[IBIS Ver]   3.2
[File Name]   sprm117a.ibs
[File Rev]   0.2
[Date]   April 12, 2004
[Source]   File Originated at Texas Instruments
[Disclaimer]   Please be aware that in the absence of a written agreement
|   Texas Instruments(TI) assumes no liability for:
|   (1) The accuracy of the IBIS models provided to your company
|   (2) The proper functioning of these Models in your design
|   or for any resulting applications;or
|   (3) Infringement of patents,copyrights, or intellectual
|   property rights resulting from your use of these models.
|   TI provides IBIS Models as a service to our customers and
|   therefore reserves the right to limit distribution of the
|   Models.
[Copyright]   Property of Texas Instruments Incorporated.
|   Unauthorized reproduction and/or distribution is strictly
|   prohibited.
|   This product is protected under copyright law and trade
|   secret law as an unpublished work.
|   Created 1999,(C) Copyright 1999-2000,
|   Texas Instruments Incorporated., All Rights Reserved.
|   These commodities are under the U.S.
|   Government distribution license control.As such,they are not
|   to be re-exported without the prior approval of the U.S.
|   Department of Commerce.
[Notes]   Includes package and IO buffer models for 1.1 and 2.0 SI.
|   REVISION HISTORY
|  Update for April 12, 2004
|   The package model and IBIS models included in this file (sprm117a)
|   apply to TMS silicon for both silcon revision 1.1 and silicon
|   revision 2.0.
|   The package model and IBIS models included in sprm117a are unchanged
|   from those models provided in sprm117.
[Component]   c6411_GLZ
[Manufacturer]   Texas Instruments
[Package]
|Variable   Typ   Min   Max
R_pkg		2.212e-01	1.101e-01	3.279e-01
L_pkg		4.011e-09	2.375e-09	5.798e-09
C_pkg		6.351e-13	3.910e-13	9.306e-13
[Pin] signal_name		model_name	R_pin		L_pin		C_pin
| Clock/PLL Configuration Section
   H4   CLKIN   IDH09_PE100   1.801e-01	3.100e-09	6.130e-13
  AE6	CLKOUT4_GP1	  IDH04_UOT335_PE100	2.381e-01	4.630e-09	6.473e-13
  AD6	CLKOUT6_GP2	  IDH04_UOT335_PE100	2.343e-01	3.341e-09	7.539e-13
   G1   RSV   NC   NA   NA   NA
   H2	  CLKMODE0   IDH09_PE100   2.283e-01	3.995e-09	6.603e-13
| JTAG Emulation Section
 AB16   TMS   IDH09_PS100   1.377e-01	2.655e-09	4.925e-13
 AE19   TDO   IDH04_OUK83_PS100	2.511e-01	4.874e-09	6.498e-13
 AF18   TDI   IDH09_PS100   2.614e-01	5.224e-09	6.920e-13
 AF16   TCLK   IDH09_PS100   2.614e-01	5.224e-09	6.920e-13
 AB15   nTRST   IDH09_PE100   2.614e-01	5.224e-09	6.920e-13
 AE18   EMU9	  IDH04_UOT335_PS100	2.477e-01	4.401e-09	6.871e-13
 AC17   EMU8	  IDH04_UOT335_PS100	1.709e-01	3.536e-09	5.334e-13
 AF17   EMU7	  IDH04_UOT335_PS100	2.500e-01	5.062e-09	6.512e-13
 AD17   EMU6	  IDH04_UOT335_PS100	1.890e-01	3.826e-09	4.936e-13
 AE17   EMU5	  IDH04_UOT335_PS100	2.341e-01	4.430e-09	6.507e-13
 AC16   EMU4	  IDH04_UOT335_PS100	1.551e-01	2.968e-09	5.512e-13
 AD16   EMU3	  IDH04_UOT335_PS100	1.987e-01	3.671e-09	6.373e-13
 AE16   EMU2	  IDH04_UOT335_PS100	2.124e-01	3.853e-09	6.090e-13
 AC15   EMU1	  IDH04_UOT335_PS100	1.646e-01	3.085e-09	5.799e-13
 AF15   EMU0	  IDH04_UOT335_PS100	2.591e-01	4.625e-09	6.938e-13
 AC18   EMU11	  IDH04_UOT335_PS100	1.860e-01	3.449e-09	5.618e-13
 AD18   EMU10	  IDH04_UOT335_PS100	2.025e-01	3.878e-09	5.902e-13
| Resets, Interrupts, and General-Purpose IOs
  AC7   nRESET   IDH09	2.025e-01	3.878e-09	5.902e-13
   B4   NMI   IDH09_PE100   2.697e-01	4.485e-09	7.472e-13
  AF4	GP7_EXTINT7   IDH04_OUK83_PS100	2.697e-01	4.485e-09	7.472e-13
  AD5	GP6_EXTINT6   IDH04_OUK83_PS100	2.697e-01	4.485e-09	7.472e-13
  AE5	GP5_EXTINT5   IDH04_OUK83_PS100	2.697e-01	4.485e-09	7.472e-13
  AF5	GP4_EXTINT4   IDH04_OUK83_PS100	2.697e-01	4.485e-09	7.472e-13
   G3	GP15_nPRST   IDI01_OUG8B	2.697e-01	4.485e-09	7.472e-13
   F2	 GP14_PCLK   IDI01_OUG8B	2.546e-01	4.449e-09	7.097e-13
   G4	GP13_nPINTA   IDI01_OUG8B	2.546e-01	4.449e-09	7.097e-13
   J3	GP12_nPGNT   IDI01_OUG8B	2.546e-01	4.449e-09	7.097e-13
   F1	GP11_nPREQ   IDI01_OUG8B	2.546e-01	4.449e-09	7.097e-13
   L2	GP10_nPCBE3   IDI01_OUG8B	2.546e-01	4.449e-09	7.097e-13
   M3	GP9_PIDSEL   IDI01_OUG8B	1.917e-01	3.882e-09	5.354e-13
  AC6   GP3   IDH04_OUK83_PE100	1.851e-01	3.359e-09	6.075e-13
  AF6   GP0   IDH04_OUK83_PE100	2.922e-01	4.494e-09	8.253e-13
  AE4   GP8   IDH04_OUK83_PE100	2.815e-01	4.759e-09	7.525e-13
| Host-Port Interface (HPI) and Peripheral Component Interconnect (PCI)
  AA4   PCIEN   IDH09_PE100   2.922e-01	4.494e-09	8.253e-13
   R4	nHINT_nPFRAME   IDI01_OUG8B	2.922e-01	4.494e-09	8.253e-13
   R1	HCNTL1_nPDEVSEL   IDI01_OUG8B	2.602e-01	4.276e-09	7.238e-13
   T4	HCNTL0_nPSTOP   IDI01_OUG8B	1.544e-01	3.008e-09	5.439e-13
   R3	HHWIL_nPTRDY   IDI01_OUG8B	1.544e-01	3.008e-09	5.439e-13
   P1	HR/nW_nPCBE2   IDI01_OUG8B	1.544e-01	3.008e-09	5.439e-13
   T3	 nHAS_PPAR   IDI01_OUG8B	1.544e-01	3.008e-09	5.439e-13
   R2	nHCS_nPPERR   IDI01_OUG8B	1.544e-01	3.008e-09	5.439e-13
   T1	nHDS1_nPSERR   IDI01_OUG8B	1.544e-01	3.008e-09	5.439e-13
   T2	nHDS2_nPCBE1   IDI01_OUG8B	1.544e-01	3.008e-09	5.439e-13
   P4	nHRDY_nPIRDY   IDI01_OUG8B	1.432e-01	2.812e-09	4.868e-13
   J2	 HD31_AD31   IDI01_OUG8B	2.239e-01	3.881e-09	6.413e-13
   K3	 HD30_AD30   IDI01_OUG8B	2.011e-01	3.696e-09	5.567e-13
   J1	 HD29_AD29   IDI01_OUG8B	2.725e-01	4.920e-09	7.166e-13
   K4	 HD28_AD28   IDI01_OUG8B	1.590e-01	3.038e-09	5.268e-13
   K2	 HD27_AD27   IDI01_OUG8B	2.196e-01	4.083e-09	6.214e-13
   L3	 HD26_AD26   IDI01_OUG8B	1.822e-01	3.378e-09	5.755e-13
   K1	 HD25_AD25   IDI01_OUG8B	2.676e-01	5.238e-09	6.857e-13
   L4	 HD24_AD24   IDI01_OUG8B	1.692e-01	3.003e-09	5.620e-13
   L1	 HD23_AD23   IDI01_OUG8B	2.646e-01	4.791e-09	6.858e-13
   M4	 HD22_AD22   IDI01_OUG8B	1.455e-01	2.797e-09	5.032e-13
   M2	 HD21_AD21   IDI01_OUG8B	2.098e-01	3.830e-09	5.948e-13
   N4	 HD20_AD20   IDI01_OUG8B	1.611e-01	2.974e-09	5.102e-13
   M1	 HD19_AD19   IDI01_OUG8B	2.475e-01	4.493e-09	6.660e-13
   N5	 HD18_AD18   IDI01_OUG8B	1.114e-01	2.452e-09	4.378e-13
   N1	 HD17_AD17   IDI01_OUG8B	2.536e-01	4.462e-09	6.731e-13
   P5	 HD16_AD16   IDI01_OUG8B	1.387e-01	2.604e-09	5.119e-13
   U4	 HD15_AD15   IDI01_OUG8B	1.709e-01	3.367e-09	5.453e-13
   U1	 HD14_AD14   IDI01_OUG8B	2.504e-01	4.977e-09	6.598e-13
   U3	 HD13_AD13   IDI01_OUG8B	1.886e-01	3.777e-09	4.994e-13
   U2	 HD12_AD12   IDI01_OUG8B	2.321e-01	4.441e-09	6.047e-13
   V4	 HD11_AD11   IDI01_OUG8B	1.869e-01	3.381e-09	5.890e-13
   V1	 HD10_AD10   IDI01_OUG8B	2.598e-01	5.197e-09	6.873e-13
   V3	 HD09_AD09   IDI01_OUG8B	2.598e-01	5.197e-09	6.873e-13
   V2	 HD08_AD08   IDI01_OUG8B	2.598e-01	5.197e-09	6.873e-13
   W2	 HD07_AD07   IDI01_OUG8B	2.598e-01	5.197e-09	6.873e-13
   W4	 HD06_AD06   IDI01_OUG8B	2.598e-01	5.197e-09	6.873e-13
   Y1	 HD05_AD05   IDI01_OUG8B	2.598e-01	5.197e-09	6.873e-13
   Y3	 HD04_AD04   IDI01_OUG8B	2.598e-01	5.197e-09	6.873e-13
   Y2	 HD03_AD03   IDI01_OUG8B	2.598e-01	5.197e-09	6.873e-13
   Y4	 HD02_AD02   IDI01_OUG8B	2.598e-01	5.197e-09	6.873e-13
  AA1	 HD01_AD01   IDI01_OUG8B	2.598e-01	5.197e-09	6.873e-13
  AA3	 HD00_AD00   IDI01_OUG8B	2.598e-01	5.197e-09	6.873e-13
   W3   nPCBE0   IDI01_OUG8B	2.598e-01	5.197e-09	6.873e-13
  AD1   XSPCS   IDH04_OUK83_PE100	2.598e-01	5.197e-09	6.873e-13
  AC2   XSPCLK   IDH04_OUK83_PE100	2.690e-01	4.510e-09	7.463e-13
  AB3   XSPDI   IDH04_PS100	2.430e-01	4.177e-09	6.584e-13
  AA2   XSPDO   IDH04_OUK83_PS100	2.703e-01	4.736e-09	7.142e-13
| EMIF Control Signals
  L26   nCE3	  IDH04_UOT335_PS100	2.598e-01	5.197e-09	6.873e-13
  K23   nCE2	  IDH04_UOT335_PS100	2.598e-01	5.197e-09	6.873e-13
  K24   nCE1	  IDH04_UOT335_PS100	2.598e-01	5.197e-09	6.873e-13
  K25   nCE0	  IDH04_UOT335_PS100	2.598e-01	5.197e-09	6.873e-13
  T23   RSV   NC   NA   NA   NA
  T24   RSV   NC   NA   NA   NA
  R25   RSV   NC   NA   NA   NA
  R26   RSV   NC   NA   NA   NA
  M25   nBE03	  IDH04_UOT335_PS100	2.598e-01	5.197e-09	6.873e-13
  M26   nBE02	  IDH04_UOT335_PS100	2.598e-01	5.197e-09	6.873e-13
  L23   nBE01	  IDH04_UOT335_PS100	2.598e-01	5.197e-09	6.873e-13
  L24   nBE00	  IDH04_UOT335_PS100	2.598e-01	5.197e-09	6.873e-13
  M22   nPDT	  IDH04_UOT335_PS100	2.598e-01	5.197e-09	6.873e-13
| EMIF Bus Arbitration
  N22   nHOLDA	  IDH04_UOT335_PS100	2.598e-01	5.197e-09	6.873e-13
  V23   nHOLD   IDH09_PS100   2.598e-01	5.197e-09	6.873e-13
  P22	  BUSREQ0	  IDH04_UOT335_PS100	2.598e-01	5.197e-09	6.873e-13
| EMIF Async/Sync Memory Control
  H25   ECLKIN   IDH09_PE100   2.511e-01	4.592e-09	6.768e-13
  J23	 ECLKOUT2	  IDH04_UOT335_PE100	1.851e-01	3.434e-09	5.608e-13
  J26	 ECLKOUT1	  IDH04_UOT335_PE100	2.599e-01	5.229e-09	6.780e-13
  J25   nSDCAS	  IDH04_UOT335_PS100	2.467e-01	4.341e-09	6.879e-13
  J24   nSDRAS	  IDH04_UOT335_PS100	2.014e-01	3.844e-09	5.854e-13
  K26   nSDWE	  IDH04_UOT335_PS100	2.494e-01	5.112e-09	6.385e-13
  L25   SDCKE	  IDH04_UOT335_PS100	2.118e-01	3.884e-09	5.955e-13
  R22   nSOE3	  IDH04_UOT335_PS100	2.118e-01	3.884e-09	5.955e-13
  L22   ARDY   IDH09_PS100   1.370e-01	2.710e-09	4.841e-13
| EMIF Address
  T22   EA22	  IDH04_UOT335_PE100	1.229e-01	2.684e-09	4.276e-13
  V24   EA21	  IDH04_UOT335_PE100	2.064e-01	3.768e-09	6.312e-13
  V25   EA20	  IDH04_UOT335_PE100	2.195e-01	4.186e-09	6.132e-13
  V26   EA19	  IDH04_UOT335_PE100	2.732e-01	4.782e-09	7.055e-13
  U23   EA18	  IDH04_UOT335_PE100	1.584e-01	2.852e-09	5.393e-13
  U24   EA17	  IDH04_UOT335_PE100	2.008e-01	3.829e-09	5.212e-13
  U25   EA16	  IDH04_UOT335_PE100	2.141e-01	4.207e-09	5.706e-13
  U26   EA15	  IDH04_UOT335_PE100	2.663e-01	5.219e-09	6.884e-13
  T25   EA14	  IDH04_UOT335_PE100	2.291e-01	3.977e-09	6.514e-13
  T26   EA13	  IDH04_UOT335_PE100	2.614e-01	4.919e-09	6.730e-13
  R23   EA12	  IDH04_UOT335_PE100	1.480e-01	3.031e-09	5.090e-13
  R24   EA11	  IDH04_UOT335_PE100	1.952e-01	3.745e-09	6.090e-13
  P23   EA10	  IDH04_UOT335_PE100	1.599e-01	3.076e-09	4.973e-13
  P24   EA09	  IDH04_UOT335_PE100	1.599e-01	3.076e-09	4.973e-13
  P26   EA08	  IDH04_UOT335_PE100	1.599e-01	3.076e-09	4.973e-13
  N23   EA07	  IDH04_UOT335_PE100	1.599e-01	3.076e-09	4.973e-13
  N24   EA06	  IDH04_UOT335_PE100	1.599e-01	3.076e-09	4.973e-13
  N26   EA05	  IDH04_UOT335_PE100	1.599e-01	3.076e-09	4.973e-13
  M23   EA04	  IDH04_UOT335_PE100	1.599e-01	3.076e-09	4.973e-13
  M24   EA03	  IDH04_UOT335_PE100	1.599e-01	3.076e-09	4.973e-13
| Reserved
 AF24   RSV   NC   NA   NA   NA
 AF23   RSV   NC   NA   NA   NA
 AE23   RSV   NC   NA   NA   NA
 AE22   RSV   NC   NA   NA   NA
 AD22   RSV   NC   NA   NA   NA
 AF22   RSV   NC   NA   NA   NA
 AD21   RSV   NC   NA   NA   NA
 AE21   RSV   NC   NA   NA   NA
 AC21   RSV   NC   NA   NA   NA
 AF21   RSV   NC   NA   NA   NA
 AD20   RSV   NC   NA   NA   NA
 AE20   RSV   NC   NA   NA   NA
 AC20   RSV   NC   NA   NA   NA
 AF20   RSV   NC   NA   NA   NA
 AC19   RSV   NC   NA   NA   NA
 AD19   RSV   NC   NA   NA   NA
  W24   RSV   NC   NA   NA   NA
  W23   RSV   NC   NA   NA   NA
  Y26   RSV   NC   NA   NA   NA
  Y23   RSV   NC   NA   NA   NA
  Y25   RSV   NC   NA   NA   NA
  Y24   RSV   NC   NA   NA   NA
 AA26   RSV   NC   NA   NA   NA
 AA23   RSV   NC   NA   NA   NA
 AA25   RSV   NC   NA   NA   NA
 AA24   RSV   NC   NA   NA   NA
 AB26   RSV   NC   NA   NA   NA
 AB24   RSV   NC   NA   NA   NA
 AB25   RSV   NC   NA   NA   NA
 AC25   RSV   NC   NA   NA   NA
 AC26   RSV   NC   NA   NA   NA
 AD26   RSV   NC   NA   NA   NA
 | EMIF Data
  C26   ED31	  IDH04_UOT335_PS100	3.097e-01	5.406e-09	7.617e-13
  D26   ED30	  IDH04_UOT335_PS100	3.225e-01	5.517e-09	8.165e-13
  D25   ED29	  IDH04_UOT335_PS100	2.683e-01	4.604e-09	7.287e-13
  E25   ED28	  IDH04_UOT335_PS100	2.825e-01	4.968e-09	7.318e-13
  E24   ED27	  IDH04_UOT335_PS100	2.414e-01	4.280e-09	6.457e-13
  E26   ED26	  IDH04_UOT335_PS100	2.953e-01	5.146e-09	7.737e-13
  F24   ED25	  IDH04_UOT335_PS100	2.271e-01	4.100e-09	5.755e-13
  F25   ED24	  IDH04_UOT335_PS100	2.711e-01	4.743e-09	7.222e-13
  F23   ED23	  IDH04_UOT335_PS100	2.131e-01	3.580e-09	6.337e-13
  F26   ED22	  IDH04_UOT335_PS100	2.841e-01	5.079e-09	7.359e-13
  G24   ED21	  IDH04_UOT335_PS100	2.217e-01	4.037e-09	6.338e-13
  G25   ED20	  IDH04_UOT335_PS100	2.556e-01	4.841e-09	6.769e-13
  G23   ED19	  IDH04_UOT335_PS100	2.034e-01	3.544e-09	6.297e-13
  G26   ED18	  IDH04_UOT335_PS100	2.698e-01	4.780e-09	7.327e-13
  H23   ED17	  IDH04_UOT335_PS100	1.904e-01	3.427e-09	5.839e-13
  H24   ED16	  IDH04_UOT335_PS100	2.066e-01	3.899e-09	5.834e-13
  C19   ED15	  IDH04_UOT335_PS100	2.140e-01	3.969e-09	6.377e-13
  D19   ED14	  IDH04_UOT335_PS100	1.703e-01	3.235e-09	5.662e-13
  A20   ED13	  IDH04_UOT335_PS100	2.811e-01	4.710e-09	7.445e-13
  D20   ED12	  IDH04_UOT335_PS100	1.756e-01	3.477e-09	5.767e-13
  B20   ED11	  IDH04_UOT335_PS100	2.338e-01	4.170e-09	6.537e-13
  C20   ED10	  IDH04_UOT335_PS100	2.189e-01	3.889e-09	6.502e-13
  A21   ED09	  IDH04_UOT335_PS100	2.189e-01	3.889e-09	6.502e-13
  D21   ED08	  IDH04_UOT335_PS100	2.189e-01	3.889e-09	6.502e-13
  B21   ED07	  IDH04_UOT335_PS100	2.189e-01	3.889e-09	6.502e-13
  C21   ED06	  IDH04_UOT335_PS100	2.189e-01	3.889e-09	6.502e-13
  A22   ED05	  IDH04_UOT335_PS100	2.189e-01	3.889e-09	6.502e-13
  C22   ED04	  IDH04_UOT335_PS100	2.189e-01	3.889e-09	6.502e-13
  B22   ED03	  IDH04_UOT335_PS100	2.189e-01	3.889e-09	6.502e-13
  B23   ED02	  IDH04_UOT335_PS100	2.189e-01	3.889e-09	6.502e-13
  A23   ED01	  IDH04_UOT335_PS100	2.189e-01	3.889e-09	6.502e-13
  A24   ED00	  IDH04_UOT335_PS100	2.189e-01	3.889e-09	6.502e-13
| Reserved pins
  A13   RSV   NC   NA   NA   NA
  C12   RSV   NC   NA   NA   NA
  B12   RSV   NC   NA   NA   NA
  A12   RSV   NC   NA   NA   NA
  D13   RSV   NC   NA   NA   NA
  C13   RSV   NC   NA   NA   NA
  E12   RSV   NC   NA   NA   NA
  E13   RSV   NC   NA   NA   NA
  B19   RSV   NC   NA   NA   NA
  E14   RSV   NC   NA   NA   NA
  A11   RSV   NC   NA   NA   NA
  D11   RSV   NC   NA   NA   NA
  D12   RSV   NC   NA   NA   NA
  A10   RSV   NC   NA   NA   NA
  B11   RSV   NC   NA   NA   NA
  C11   RSV   NC   NA   NA   NA
  E15   RSV   NC   NA   NA   NA
  E11   RSV   NC   NA   NA   NA
  D17   RSV   NC   NA   NA   NA
  C17   RSV   NC   NA   NA   NA
  A17   RSV   NC   NA   NA   NA
  D16   RSV   NC   NA   NA   NA
  C16   RSV   NC   NA   NA   NA
  B16   RSV   NC   NA   NA   NA
  A16   RSV   NC   NA   NA   NA
  D15   RSV   NC   NA   NA   NA
  C15   RSV   NC   NA   NA   NA
  B15   RSV   NC   NA   NA   NA
  A15   RSV   NC   NA   NA   NA
  D14   RSV   NC   NA   NA   NA
  C14   RSV   NC   NA   NA   NA
  A14   RSV   NC   NA   NA   NA
   D7   RSV   NC   NA   NA   NA
   B6   RSV   NC   NA   NA   NA
   C7   RSV   NC   NA   NA   NA
   A6   RSV   NC   NA   NA   NA
   D8   RSV   NC   NA   NA   NA
   B7   RSV   NC   NA   NA   NA
   C8   RSV   NC   NA   NA   NA
   A7   RSV   NC   NA   NA   NA
   C9   RSV   NC   NA   NA   NA
   B8   RSV   NC   NA   NA   NA
   D9   RSV   NC   NA   NA   NA
   B9   RSV   NC   NA   NA   NA
  C10   RSV   NC   NA   NA   NA
   A9   RSV   NC   NA   NA   NA
  D10   RSV   NC   NA   NA   NA
  B10   RSV   NC   NA   NA   NA
|Device Configuration
  E16   LEND	  IDH04_UOT335_PS100	1.226e-01	2.604e-09	4.665e-13
  D18   BOOTMODE1	  IDH04_UOT335_PS100	1.641e-01	2.969e-09	5.594e-13
  C18   BOOTMODE0	  IDH04_UOT335_PE100	2.067e-01	3.758e-09	6.201e-13
  B18   ECLKIN_SEL1  IDH04_UOT335_PE100	2.194e-01	4.208e-09	6.099e-13
  A18   ECLKIN_SEL0  IDH04_UOT335_PE100	2.767e-01	5.325e-09	6.838e-13
  B17   EEAI	  IDH04_UOT335_PE100	2.141e-01	4.201e-09	5.714e-13
| Timer 2
   A4   TOUT2   IDH04_OUK83_PE100	3.211e-01	5.798e-09	7.928e-13
   C5   TINP2   IDH09_PE100   2.423e-01	4.149e-09	6.777e-13
| Timer 1
   B5   TOUT1   IDH04_OUK83_PE100	2.850e-01	4.720e-09	7.582e-13
   A5   TINP1   IDH09_PE100   2.956e-01	5.023e-09	7.720e-13
| Timer 0
   D6   TOUT0   IDH04_OUK83_PE100	2.113e-01	3.835e-09	6.281e-13
   C6   TINP0   IDH09_PE100   2.266e-01	4.066e-09	6.171e-13
| Reserved
  AF3   RSV   NC   NA   NA   NA
  AB1   RSV   NC   NA   NA   NA
  AC1   RSV   NC   NA   NA   NA
  AB2   RSV   NC   NA   NA   NA
| MultiChannel Buffered Serial Port 1 (McBSP1)
  AC8   CLKS1   IDH04_OUK83	1.696e-01	3.371e-09	5.336e-13
 AC10   CLKR1   IDH04_OUK83	1.577e-01	2.917e-09	5.345e-13
 AB12   CLKX1   IDH04_OUK83	1.314e-01	2.568e-09	4.920e-13
 AF11   DR1   IDH04_OUK83	2.619e-01	4.872e-09	6.818e-13
 AB11   DX1   IDH04_OUK83	1.224e-01	2.641e-09	4.477e-13
  AC9   FSR1   IDH04_OUK83	1.641e-01	2.958e-09	5.482e-13
 AB13   FSX1   IDH04_OUK83	1.112e-01	2.390e-09	4.431e-13
| MultiChannel Buffered Serial Port 0 (McBSP0)
   F4   CLKS0   IDH09_PE100   1.913e-01	3.477e-09	6.149e-13
   D1   CLKR0   IDH04_OUK83_PE100	2.976e-01	5.157e-09	7.602e-13
   E1   CLKX0   IDH04_OUK83_PE100	3.080e-01	5.297e-09	7.859e-13
   D2   DR0   IDH04_PS100	2.825e-01	4.838e-09	7.380e-13
   E2   DX0   IDH04_OUK83_PS100	2.580e-01	4.588e-09	6.760e-13
   C1   FSR0   IDH04_OUK83_PE100	3.009e-01	4.906e-09	7.948e-13
   E3   FSX0   IDH04_OUK83_PE100	2.445e-01	4.090e-09	6.962e-13
|Reserved
 AD11   RSV   NC   NA   NA   NA
 AC14   RSV   NC   NA   NA   NA
 AE15   RSV   NC   NA   NA   NA
 AC13   RSV   NC   NA   NA   NA
  AE9   RSV   NC   NA   NA   NA
 AD10   RSV   NC   NA   NA   NA
  AD9   RSV   NC   NA   NA   NA
  AD8   RSV   NC   NA   NA   NA
  AE8   RSV   NC   NA   NA   NA
  AF9   RSV   NC   NA   NA   NA
  AF7   RSV   NC   NA   NA   NA
  AE7   RSV   NC   NA   NA   NA
  AD7   RSV   NC   NA   NA   NA
 AD12   RSV   NC   NA   NA   NA
 AF14   RSV   NC   NA   NA   NA
 AD15   RSV   NC   NA   NA   NA
 AB14   RSV   NC   NA   NA   NA
 AF10   RSV   NC   NA   NA   NA
 AE10   RSV   NC   NA   NA   NA
 AF12   RSV   NC   NA   NA   NA
 AE11   RSV   NC   NA   NA   NA
 AF13   RSV   NC   NA   NA   NA
 AC11   RSV   NC   NA   NA   NA
 AC12   RSV   NC   NA   NA   NA
 AE12   RSV   NC   NA   NA   NA
 AD14   RSV   NC   NA   NA   NA
 AD13   RSV   NC   NA   NA   NA
| End of Package Model
[Component]   IDH04_UOT335_PE100
[Manufacturer]   Texas Instruments
[Package]
|   typ   min   max
R_pkg   0   0   0
L_pkg   0   0   0
C_pkg   0   0   0
[Pin]   signal_name   model_name   R_pin   L_pin   C_pin
   1   Y  IDH04_UOT335_PE100   0   0   0
[Component]   IDH04_PS100
[Manufacturer]   Texas Instruments
[Package]
|   typ   min   max
R_pkg   0   0   0
L_pkg   0   0   0
C_pkg   0   0   0
[Pin]   signal_name   model_name   R_pin   L_pin   C_pin
   1   A   IDH04_PS100   0   0   0
[Component]   IDH04_OUK83_PS100
[Manufacturer]   Texas Instruments
[Package]
|   typ   min   max
R_pkg   0   0   0
L_pkg   0   0   0
C_pkg   0   0   0
[Pin]   signal_name   model_name   R_pin   L_pin   C_pin
   1   Y   IDH04_OUK83_PS100   0   0   0
[Component]   IDH04_UOT335_PS100
[Manufacturer]   Texas Instruments
[Package]
|   typ   min   max
R_pkg   0   0   0
L_pkg   0   0   0
C_pkg   0   0   0
[Pin]   signal_name   model_name   R_pin   L_pin   C_pin
   1   Y  IDH04_UOT335_PS100   0   0   0
[Component]   IDH09
[Manufacturer]   Texas Instruments
[Package]
|   typ   min   max
R_pkg   0   0   0
L_pkg   0   0   0
C_pkg   0   0   0
[Pin]   signal_name   model_name   R_pin   L_pin   C_pin
   1   A   IDH09   0   0   0
[Component]   IDH09_PS100
[Manufacturer]   Texas Instruments
[Package]
|   typ   min   max
R_pkg   0   0   0
L_pkg   0   0   0
C_pkg   0   0   0
[Pin]   signal_name   model_name   R_pin   L_pin   C_pin
   1   A   IDH09_PS100   0   0   0
[Component]   IDH09_PE100
[Manufacturer]   Texas Instruments
[Package]
|   typ   min   max
R_pkg   0   0   0
L_pkg   0   0   0
C_pkg   0   0   0
[Pin]   signal_name   model_name   R_pin   L_pin   C_pin
   1   A   IDH09_PE100   0   0   0
[Component]   IDI01_OUG8B
[Manufacturer]   Texas Instruments
[Package]
|   typ   min   max
R_pkg   0   0   0
L_pkg   0   0   0
C_pkg   0   0   0
[Pin]   signal_name   model_name   R_pin   L_pin   C_pin
   1   Y   IDI01_OUG8B   0   0   0
[Component]   IDH04_OUK83_PE100
[Manufacturer]   Texas Instruments
[Package]
|   typ   min   max
R_pkg   0   0   0
L_pkg   0   0   0
C_pkg   0   0   0
[Pin]   signal_name   model_name   R_pin   L_pin   C_pin
   1   Y   IDH04_OUK83_PE100   0   0   0
[Component]   IDH04_OUK83
[Manufacturer]   Texas Instruments
[Package]
|   typ   min   max
R_pkg   0   0   0
L_pkg   0   0   0
C_pkg   0   0   0
[Pin]   signal_name   model_name   R_pin   L_pin   C_pin
   1   Y   IDH04_OUK83   0   0   0
| Models and submodels in the file (10): IDH04_UOT335_PE100 (I/O), IDH04_PS100 (Input), IDH04_OUK83_PS100 (I/O), IDH04_UOT335_PS100 (I/O), IDH09 (Input), IDH09_PS100 (Input), IDH09_PE100 (Input), IDI01_OUG8B (I/O), IDH04_OUK83_PE100 (I/O), IDH04_OUK83 (I/O)
